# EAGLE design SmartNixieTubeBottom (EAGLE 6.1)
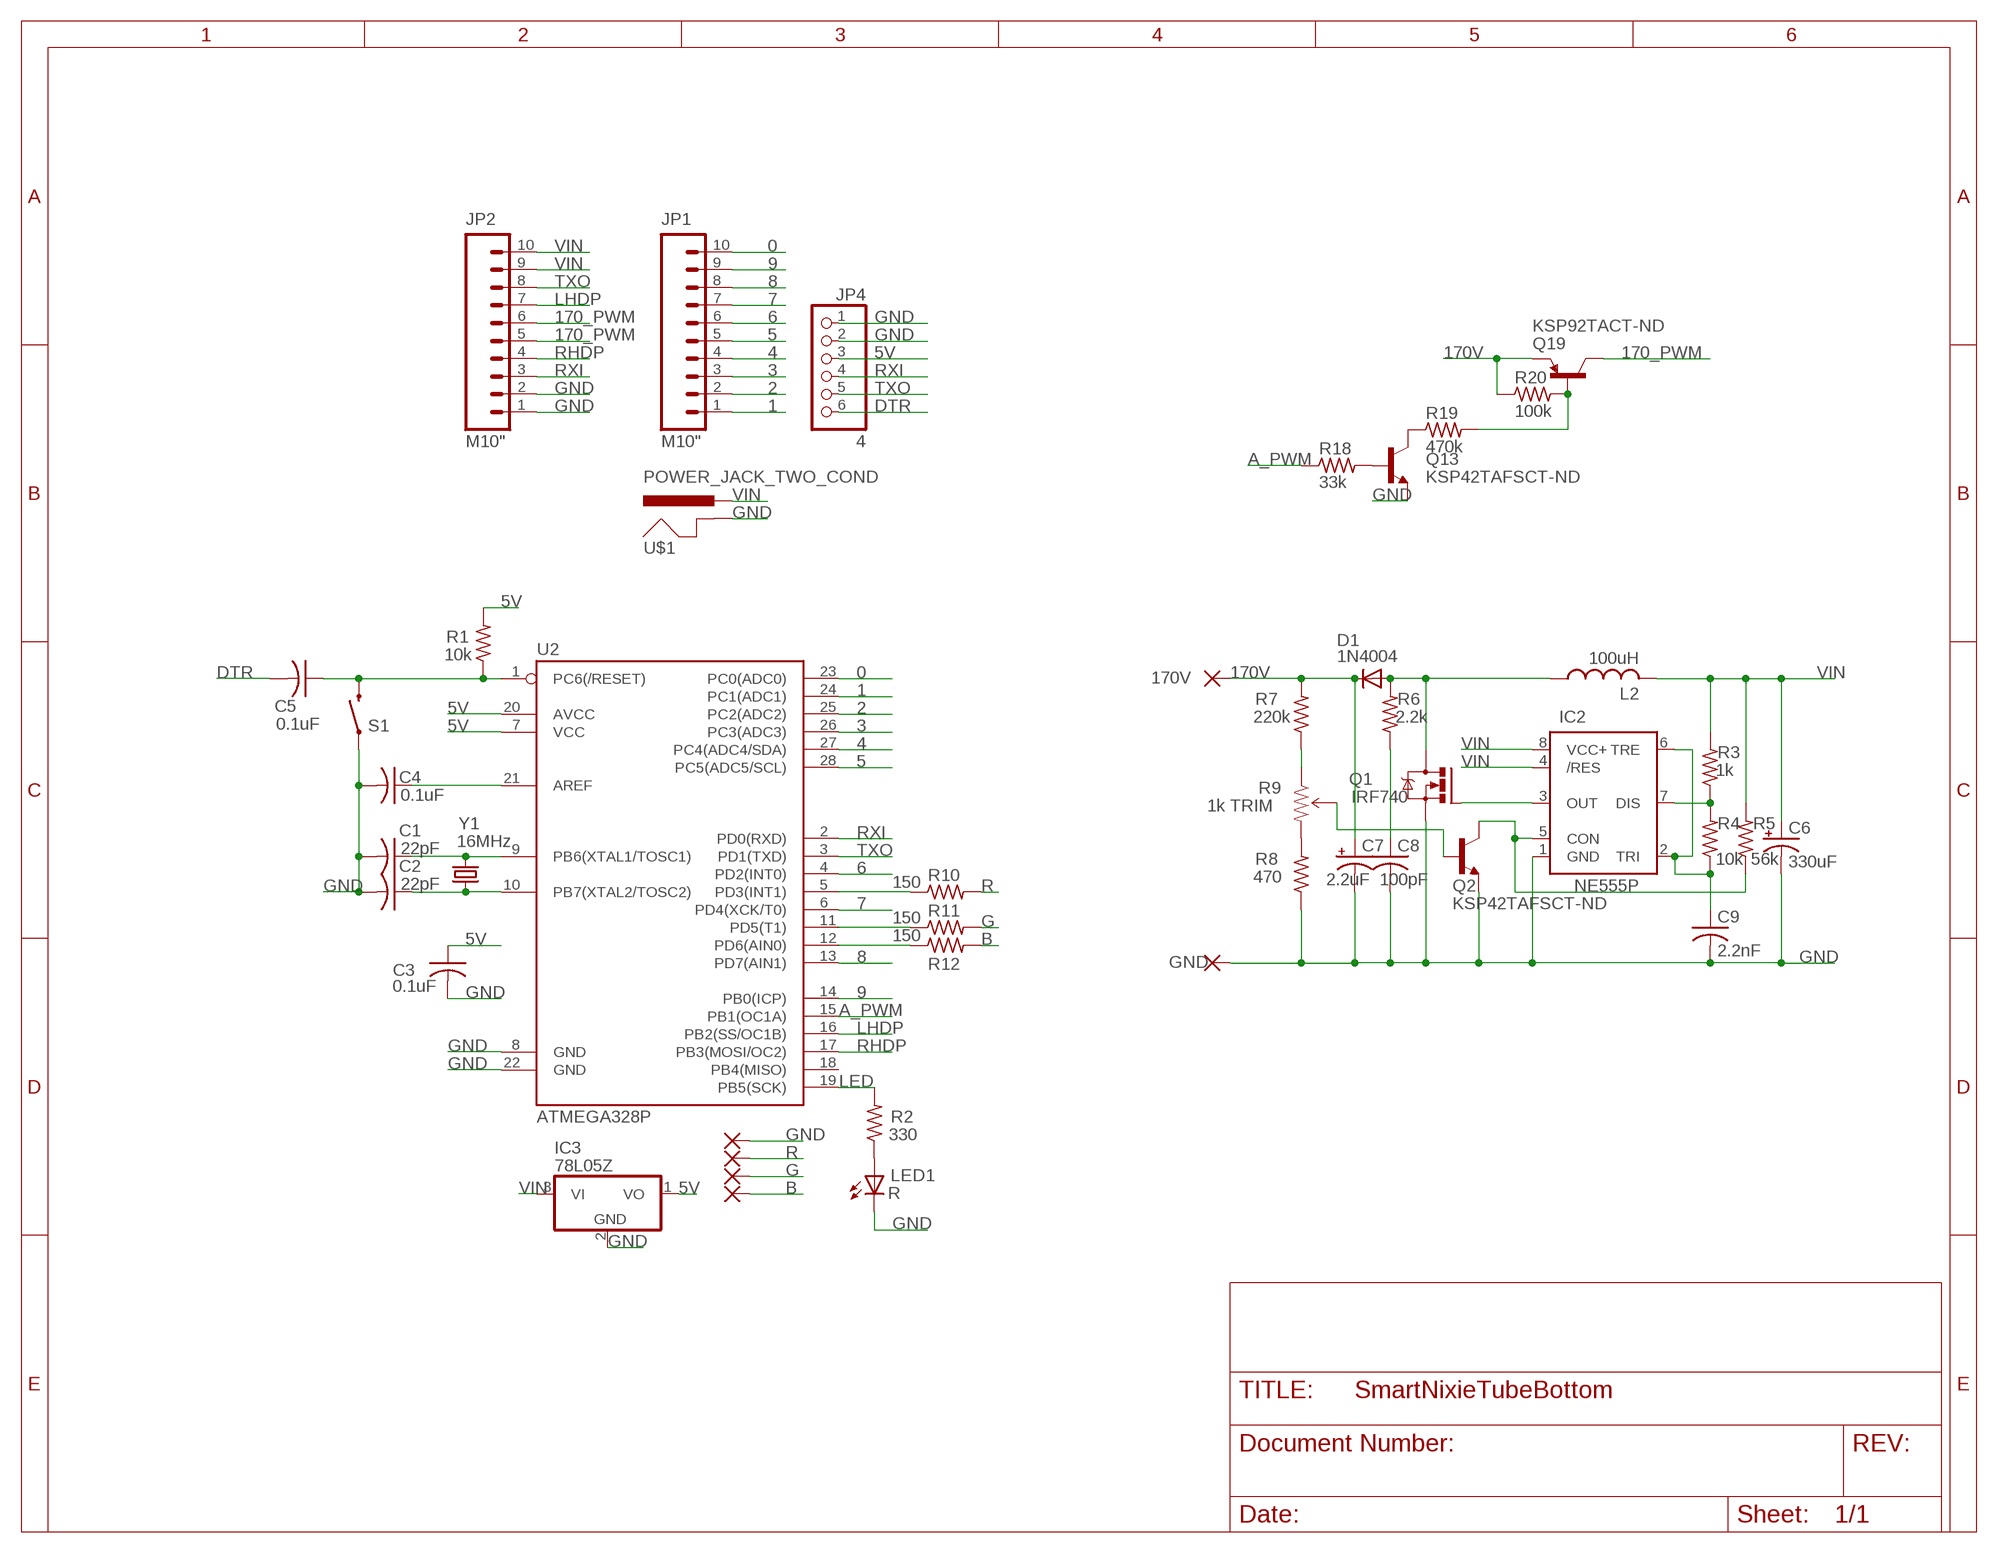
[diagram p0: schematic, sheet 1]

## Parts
C1  22pF  C-US025-024X044  [C025-024X044]
C2  22pF  C-US025-024X044  [C025-024X044]
C3  0.1uF  C-US025-024X044  [C025-024X044]
C4  0.1uF  C-US025-024X044  [C025-024X044]
C5  0.1uF  C-US025-024X044  [C025-024X044]
C6  330uF  CPOL-USE2,5-6E  [E2,5-6E]
C7  2.2uF  CPOL-USE2,5-6E  [E2,5-6E]
C8  100pF  C-US050-025X075  [C050-025X075]
C9  2.2nF  C-US025-025X050  [C025-025X050]
D1  1N4004  [DO41-10]
IC2  NE555P  [DIL-08]
IC3  78L05Z  [TO92]
JP1  M10"  [1X10]
JP2  M10"  [1X10]
JP4  4  PINHD-1X6/90  [1X06/90]
L2  100uH  L-US6000-XXX-RC  [6000-XXXX-RC]
LED1  R  LED5MM  [LED5MM]
PAD1  1  2,15/1,0  [2,15/1,0]
PAD2  2  2,15/1,0  [2,15/1,0]
PAD3  3  2,15/1,0  [2,15/1,0]
PAD4  4  2,15/1,0  [2,15/1,0]
PAD13  GND  1,6/0,8  [1,6/0,8]
PAD14  170V  1,6/0,8  [1,6/0,8]
Q1  IRF740  [TO220BV]
Q2  KSP42TAFSCT-ND  TRANSISTOR_NPNTO-92-AMMO  [TO-92-AMMO]
Q13  KSP42TAFSCT-ND  TRANSISTOR_NPNTO-92-AMMO  [TO-92-AMMO]
Q19  KSP92TACT-ND  TRANSISTOR_PNP  [TO-92-AMMO]
R1  10k  R-US_0204/5  [0204/5]
R2  330  R-US_0204/5  [0204/5]
R3  1k  R-US_0204/5  [0204/5]
R4  10k  R-US_0204/5  [0204/5]
R5  56k  R-US_0204/5  [0204/5]
R6  2.2k  R-US_0204/5  [0204/5]
R7  220k  R-US_0204/5  [0204/5]
R8  470  R-US_0204/5  [0204/5]
R9  1k TRIM  TRIMPOTPTH  [TRIM_POT_PTH]
R10  150  R-US_0204/5  [0204/5]
R11  150  R-US_0204/5  [0204/5]
R12  150  R-US_0204/5  [0204/5]
R18  33k  R-US_0204/5  [0204/5]
R19  470k  R-US_0204/5  [0204/5]
R20  100k  R-US_0204/5  [0204/5]
S1  SWITCH-MOMENTARY-2PTH  [TACTILE-PTH]
U2  ATMEGA328P  ATMEGA328P_PDIP  [DIL28-3]
U$1  POWER_JACK_TWO_COND  [POWER_JACK_TWO_COND]
Y1  16MHz  CRYSTALHC49US  [HC49US]

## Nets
0: JP1.10 U2.23(PC0(ADC0))
1: JP1.1 U2.24(PC1(ADC1))
2: JP1.2 U2.25(PC2(ADC2))
3: JP1.3 U2.26(PC3(ADC3))
4: JP1.4 U2.27(PC4(ADC4/SDA))
5: JP1.5 U2.28(PC5(ADC5/SCL))
5V: C3.1 IC3.1(VO) JP4.3 R1.2 U2.7(VCC) U2.20(AVCC)
6: JP1.6 U2.4(PD2(INT0))
7: JP1.7 U2.6(PD4(XCK/T0))
8: JP1.8 U2.13(PD7(AIN1))
9: JP1.9 U2.14(PB0(ICP))
170_PWM: JP2.5 JP2.6 Q19.3(C)
170V: C7.+ D1.C PAD14.1(P) Q19.1(E) R7.2 R20.1
A_PWM: R18.1 U2.15(PB1(OC1A))
B: PAD4.1(P) R12.2
DTR: C5.2 JP4.6
G: PAD3.1(P) R11.2
GND: C1.2 C2.2 C3.2 C4.2 C6.- C7.- C8.2 C9.2 IC2.1(GND) IC3.2(GND) JP2.1 JP2.2 JP4.1 JP4.2 LED1.K(C) PAD1.1(P) PAD13.1(P) Q1.S Q2.1(E) Q13.1(E) R8.1 S1.1 U2.8(GND) U2.22(GND) U$1.P$1(GNDBREAK)
LED: R2.2 U2.19(PB5(SCK))
LHDP: JP2.7 U2.16(PB2(SS/OC1B))
N$1: C1.1 U2.9(PB6(XTAL1/TOSC1)) Y1.2
N$2: C2.1 U2.10(PB7(XTAL2/TOSC2)) Y1.1
N$3: C4.1 U2.21(AREF)
N$4: LED1.A R2.1
N$5: IC2.3(OUT) Q1.G
N$7: IC2.7(DIS) R3.1 R4.2
N$8: C9.1 IC2.2(TRI) IC2.6(TRE) R4.1
N$9: IC2.5(CON) Q2.3(C) R5.1
N$10: D1.A L2.1 Q1.D R6.2
N$11: C8.1 R6.1
N$12: R8.2 R9.3(CW)
N$13: R7.1 R9.1(CCW)
N$14: Q2.2(B) R9.2(WIPER)
N$15: Q13.2(B) R18.2
N$17: R10.1 U2.5(PD3(INT1))
N$18: R11.1 U2.11(PD5(T1))
N$19: R12.1 U2.12(PD6(AIN0))
N$20: Q13.3(C) R19.1
N$28: Q19.2(B) R19.2 R20.2
R: PAD2.1(P) R10.2
RESET: C5.1 R1.1 S1.3 U2.1(PC6(/RESET))
RHDP: JP2.4 U2.17(PB3(MOSI/OC2))
RXI: JP2.3 JP4.4 U2.2(PD0(RXD))
TXO: JP2.8 JP4.5 U2.3(PD1(TXD))
VIN: C6.+ IC2.4(/RES) IC2.8(VCC+) IC3.3(VI) JP2.9 JP2.10 L2.2 R3.2 R5.2 U$1.P$2(PWR)
Unconnected: U2.18(PB4(MISO))

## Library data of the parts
C1-C5 C8 = rcl:C-US: CAPACITOR, American symbol
C6 C7 = resistor:CPOL-US: POLARIZED CAPACITOR, American symbol
C9 = resistor:C-US: CAPACITOR, American symbol
D1 = diode:1N4004: DIODE
IC2 = SparkFun-AnalogIC:NE555: General purpose bipolar Timer; MF: Arrow Electronics; MPN: NE555N; OC_FARNELL: 1467742; OC_NEWARK: 89K1486
IC3 = linear:78*: Positive VOLTAGE REGULATOR Source: http://cache.national.com/ds/LM/LM78L05.pdf http://www.fairchildsemi.com/ds/LM/LM7805.pdf
JP1 JP2 = SparkFun-Connectors_tyler:M10: Header 10 Standard 10-pin 0.1" header. Use with straight break away headers (SKU : PRT-00116), right angle break away headers (PRT-00553), swiss pins (PRT-00743), machine pins (PRT-00117), and female headers (PRT-00115).
JP4 = pinhead:PINHD-1X6: PIN HEADER
L2 = rcl:L-US: INDUCTOR, American symbol
LED1 = SparkFun-LED:LED: LEDs
PAD1-PAD4 = wirepad:2,15/1,0: THROUGH-HOLE PAD
PAD13 PAD14 = wirepad:1,6/0,8: THROUGH-HOLE PAD
Q1 = transistor-power:IRF740: N-CHANNEL MOS FET
Q2 Q13 = SparkFun-DiscreteSemi:TRANSISTOR_NPN: Generic NPN BJT. MMBT2222 is the common NPN we use. Double check against datasheet- not all devices are the same!
Q19 = SparkFun-DiscreteSemi_tyler:TRANSISTOR_PNP: Generic PNP BJT. Double check pinouts against datasheets- not all devices are the same!
R1-R8 R10-R12 R18-R20 = resistor:R-US_: RESISTOR, American symbol
R9 = SparkFun-Electromechanical:TRIMPOT: Various small potentiometers for "set-and-forget" applications
S1 = SparkFun-Electromechanical:SWITCH-MOMENTARY-2: Various NO switches- pushbuttons, reed, etc
U2 = SparkFun-DigitalIC_tyler:ATMEGA328P_PDIP: uC used in the Arduino 32kb flash, 1k EEPROM, 2k SRAM This is the through-hole version of this chip.
U$1 = SparkFun-Connectors_tyler:POWER_JACK_TWO_COND
Y1 = SparkFun-FreqCtrl:CRYSTAL: Various standard crystals. Proven footprints. Spark Fun Electronics SKU : COM-00534

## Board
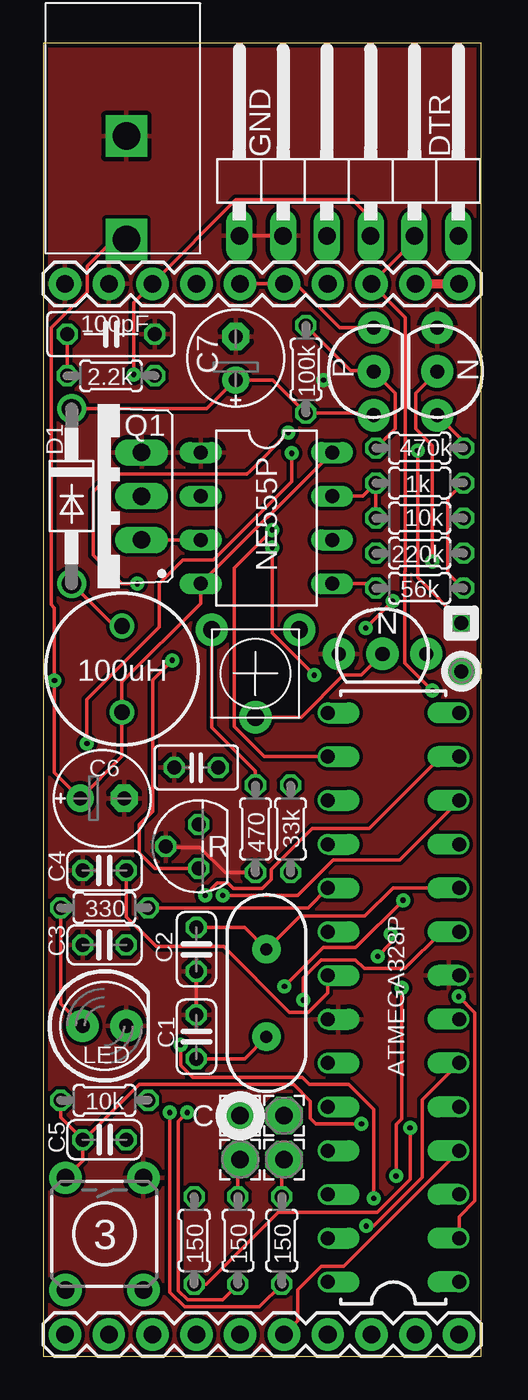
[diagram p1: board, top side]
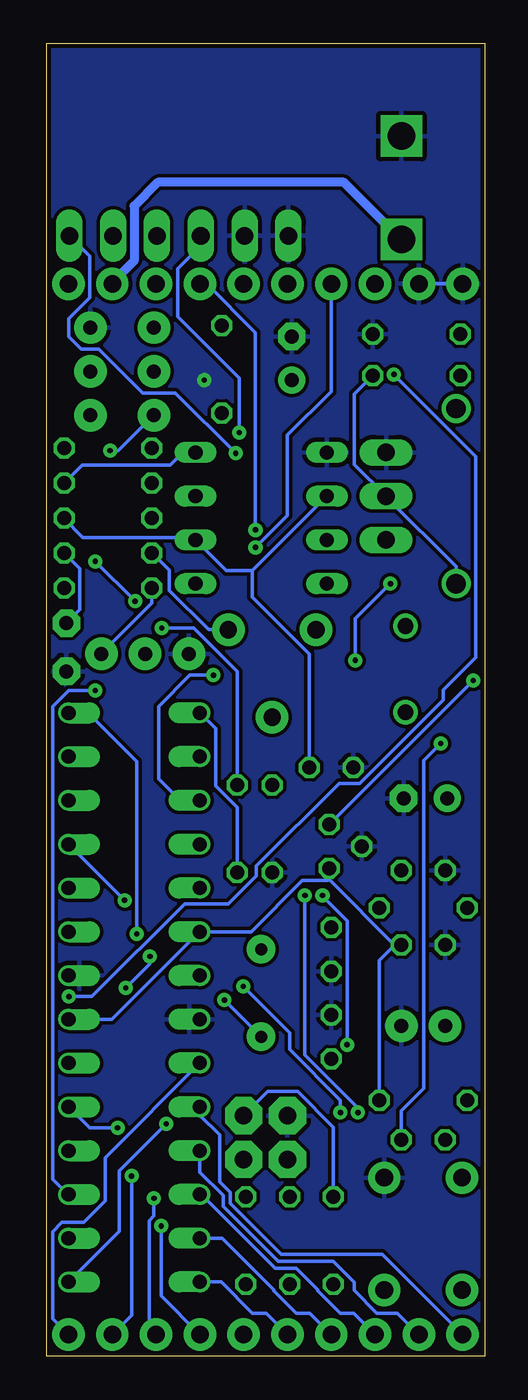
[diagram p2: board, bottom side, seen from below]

Size 25.41 x 76.2 mm. Coordinates in mm from the lower left corner, seen from the top.
Outline: 0,0 25.41,0 25.41,76.2 0,76.2 0,0
Copper layers (1*16): Top 0.035mm / dielectric 1.5mm / Bottom 0.035mm
Design rules: minimum track width 8mil, minimum drill 12mil, track to track 8mil, track to pad 8mil, pad to pad 8mil, via to via 8mil, smd to smd 8mil, copper to edge 10mil, drill to drill 6mil, minimum pad ring 8mil, minimum via ring 10mil, stop-mask expansion 4mil, vias tented up to drill 25mil, thermal gap 10mil

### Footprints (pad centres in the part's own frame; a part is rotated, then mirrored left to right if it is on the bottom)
C025-024X044 = drill 0.813 octagon: 1 -1.27,0; 2 1.27,0
E2,5-6E = drill 0.813 pad 1.575: + -1.27,0 | drill 0.813 pad 1.575 octagon: - 1.27,0
C050-025X075 = drill 0.813 octagon: 1 -2.54,0; 2 2.54,0
C025-025X050 = drill 0.813 octagon: 1 -1.27,0; 2 1.27,0
DO41-10 = drill 1.118: A 5.08,0; C -5.08,0
DIL-08 = drill 0.813 long: 1 -3.81,-3.81; 2 -1.27,-3.81; 3 1.27,-3.81; 4 3.81,-3.81; 5 3.81,3.81; 6 1.27,3.81; 7 -1.27,3.81; 8 -3.81,3.81
TO92 = drill 0.813 octagon: 1 -1.27,0; 2 0,1.905; 3 1.27,0
1X10 = drill 1.016 pad 1.88: 1 0,0; 2 2.54,0; 3 5.08,0; 4 7.62,0; 5 10.16,0; 6 12.7,0; 7 15.24,0; 8 17.78,0; 9 20.32,0; 10 22.86,0
1X06/90 = drill 1.016 long: 1 -6.35,-3.81; 2 -3.81,-3.81; 3 -1.27,-3.81; 4 1.27,-3.81; 5 3.81,-3.81; 6 6.35,-3.81
6000-XXXX-RC = drill 0.9 pad 1.422: 1 -2.5,0; 2 2.5,0
LED5MM = drill 0.813 pad 1.88: A -1.27,0; K 1.27,0
2,15/1,0 = drill 1.016 pad 2.159 octagon: 1 0,0
1,6/0,8 = drill 0.813 pad 1.6 octagon: 1 0,0
TO220BV = drill 1.016 long: D 0,-2.54; G -2.54,-2.54; S 2.54,-2.54
TO-92-AMMO = drill 0.813 pad 1.88: 1 -2.54,0; 2 0,0; 3 2.54,0
0204/5 = drill 0.813 octagon: 1 -2.54,0; 2 2.54,0
TRIM_POT_PTH = drill 1 pad 1.88: 1 -2.54,-2.54; 2 0,2.54; 3 2.54,-2.54
TACTILE-PTH = drill 1.016 pad 1.88: 1 -3.251,2.261; 2 3.251,2.261; 3 -3.251,-2.261; 4 3.251,-2.261
DIL28-3 = drill 0.813 offset: 1 -16.51,-3.81; 2 -13.97,-3.81; 3 -11.43,-3.81; 4 -8.89,-3.81; 5 -6.35,-3.81; 6 -3.81,-3.81; 7 -1.27,-3.81; 8 1.27,-3.81; 9 3.81,-3.81; 10 6.35,-3.81; 11 8.89,-3.81; 12 11.43,-3.81; 13 13.97,-3.81; 14 16.51,-3.81; 15 16.51,3.81; 16 13.97,3.81; 17 11.43,3.81; 18 8.89,3.81; 19 6.35,3.81; 20 3.81,3.81; 21 1.27,3.81; 22 -1.27,3.81; 23 -3.81,3.81; 24 -6.35,3.81; 25 -8.89,3.81; 26 -11.43,3.81; 27 -13.97,3.81; 28 -16.51,3.81
POWER_JACK_TWO_COND = drill 1.6 square: P$1 4.7,6.8; P$2 4.7,0.8
HC49US = drill 0.7 pad 1.651: 1 -2.54,0; 2 2.54,0

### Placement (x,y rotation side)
C1  8.89,18.54 90 top
C2  8.89,23.62 270 top
C3  3.56,23.88 180 top
C4  3.56,28.19 180 top
C5  3.56,12.57 0 top
C6  3.43,32.38 0 top
C7  11.18,57.91 90 top
C8  3.94,59.31 0 top
C9  8.89,34.16 180 top
D1  1.65,49.91 270 top
IC2  12.95,48.64 270 top
IC3  9.02,29.59 90 top
JP1  1.27,1.27 0 top
JP2  1.27,62.23 0 top
JP4  17.73,68.83 0 top
L2  4.57,39.88 270 top
LED1  3.56,19.18 0 top
PAD1  11.43,13.97 0 top
PAD2  13.97,13.97 0 top
PAD3  11.43,11.43 0 top
PAD4  13.97,11.43 0 top
PAD13  24.26,39.75 0 top
PAD14  24.26,42.55 0 top
Q1  3.17,49.91 90 top
Q2  19.68,40.77 0 top
Q13  22.86,57.15 270 top
Q19  19.18,57.15 90 top
R1  3.56,14.86 0 top
R2  3.56,26.04 0 top
R3  21.84,50.67 0 top
R4  21.84,48.64 180 top
R5  21.84,44.58 0 top
R6  3.94,56.9 0 top
R7  21.84,46.61 0 top
R8  12.32,30.61 90 top
R9  12.32,39.62 180 top
R10  8.76,6.73 90 top
R11  11.3,6.73 90 top
R12  13.84,6.73 90 top
R18  14.35,30.61 90 top
R19  21.84,52.7 180 top
R20  15.24,57.28 90 top
S1  3.56,7.11 270 top
U2  20.32,20.83 90 top
U$1  0.13,64.01 0 top
Y1  12.95,21.08 270 top

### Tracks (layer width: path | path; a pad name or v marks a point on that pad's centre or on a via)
0
  Bottom 0.203: U2.23 22,11.53 22,9.02 23.24,7.77 24.51,7.77 25.04,7.24 25.04,2.18 JP1.10
1
  Bottom 0.203: U2.24 16.51,13.99 15.37,12.85 15.37,10.13 14.76,9.53 14.76,8.89 11.79,5.92 5.92,5.92 JP1.1
2
  Bottom 0.203: U2.25 16.51,10.69 15.16,9.35 15.16,8.71 11.96,5.51 8.79,5.51 7.57,4.29 7.57,3.83 6.25,2.52 5.05,2.52 JP1.2
3
  Bottom 0.203: U2.26 16.43,9.4 12.14,5.11 10.92,5.11 9.68,3.86 9.68,3.81 8.38,2.52 7.59,2.52 JP1.3
4
  Bottom 0.203: U2.27 15.21,6.86 12.22,3.86 12.22,3.81 10.92,2.52 10.13,2.52 JP1.4
5
  Bottom 0.203: U2.28 15.27,4.32 13.46,2.52 12.68,2.52 JP1.5
5V  (via drill 0.3)
  Top 0.203: v14.22,53.59 12,51.37 11.81,51.18 3.94,51.18 2.92,50.16 2.92,46.48 4.57,44.83 v5.46,44.83 | IC3.1 6.48,28.32 5.59,29.21 5.59,30.86 6.35,31.62 6.35,39.24 v7.49,40.39
  Bottom 0.203: 9.02,27.66 5.23,23.88 C3.1 5.28,23.8 6.1,22.99 R1.2 | IC3.1 9.02,27.66 | 9.02,27.66 9.09,27.61 10.57,27.61 13.54,24.64 U2.20 16.59,24.59 21.61,19.56 U2.7 | JP4.3 16.46,64.44 17.78,63.12 17.78,60.33 14.22,56.77 v14.22,53.59 | v7.49,40.39 7.49,42.8 v5.46,44.83
6
  Top 0.203: U2.4 17.42,5.23 16.13,5.23 14.76,3.86 14.76,2.06 JP1.6
7  (via drill 0.3)
  Top 0.203: U2.6 22,14.88 22,10.39 19.18,7.57 v18.75,7.57
  Bottom 0.203: v18.75,7.57 18.75,3.5 JP1.7
8  (via drill 0.3)
  Top 0.203: U2.13 23.09,34.8 18.92,30.63 15.62,30.63 13.23,28.25 13.23,27.69 12.7,27.15 11.02,27.15 10.72,27.46 10.11,27.46 v9.4,26.75 | v7.98,18.09 7.98,16.89 8.69,16.18 15.04,16.18 15.44,15.77 17.73,15.77 19.18,14.33 v19.18,9.17
  Bottom 0.203: v9.4,26.75 9.4,26.7 7.98,25.27 v7.98,18.09 | v19.18,9.17 19.18,8.15 19.46,7.87 19.46,1.68 JP1.8
9  (via drill 0.3)
  Top 0.203: v20.17,24.51 20.17,23.98 v19.41,23.22 | v20.8,21.39 20.8,13.79 20.47,13.46 v20.47,10.46
  Bottom 0.203: U2.14 22.99,37.34 20.17,34.52 v20.17,24.51 | v19.41,23.22 19.41,22.78 v20.8,21.39 | v20.47,10.46 20.47,2.39 JP1.9
170_PWM
  Top 0.203: JP2.5 JP2.6 14.05,62.18 14.71,62.18 17.2,59.69 Q19.3
170V  (via drill 0.3)
  Top 0.203: Q19.1 19.05,54.74 R20.1 15.16,54.79 13.31,56.64 C7.+ 11.1,56.59 9.5,54.99 D1.C | PAD14.1 24.26,42.65 21.72,45.19 v21.72,52.55
  Bottom 0.203: R7.2 24.38,46.63 23.47,45.72 23.47,43.33 PAD14.1 | v21.72,52.55 21.23,52.55 Q19.1
A_PWM
  Bottom 0.203: R18.1 14.35,31.85 15.6,33.1 15.6,36.42 U2.15
B
  Top 0.203: R12.2 13.84,11.3 PAD4.1
DTR  (via drill 0.3)
  Top 0.203: v2.54,35.56 2.54,38.12 6.73,42.32 6.73,44.83 8.1,46.2 9.88,46.2 14.43,50.75 v14.43,52.4
  Bottom 0.203: C5.2 4.83,14.25 3.53,15.54 3.53,34.57 v2.54,35.56 | v14.43,52.4 17.93,55.91 19.84,55.91 22.38,58.45 23.39,58.45 24.11,59.16 24.11,60.22 22.89,61.44 22.89,63.83 JP4.6
G
  Top 0.203: R11.2 11.3,11.3 PAD3.1
GND  (via drill 0.3)
  Top 0.203: JP4.2 JP4.1 | R8.1 10.57,28.07 9.09,29.54 7.19,29.54 IC3.2 | C2.2 C1.2
  Bottom 0.203: JP2.2 JP2.1
  other vias: 16.26,56.64
  pour Bottom (isolate 0.203): 0,0 25.4,0 25.4,76.2 0,76.2
  pour Top (isolate 0.203): 0,0 25.4,0 25.4,76.2 0,76.2
LED
  Top 0.203: R2.2 15.37,26.04 U2.19
LHDP  (via drill 0.3)
  Top 0.203: U2.16 12.83,34.8 11.07,36.55 11.07,45.74 v13.28,47.95
  Bottom 0.203: v13.28,47.95 13.28,59.41 16.1,62.23 JP2.7
N$1  (via drill 0.3)
  Top 0.203: C1.1 11.68,17.27 Y1.2 | U2.9 23.11,24.64 20.98,22.5 18.62,22.5 18.11,23.01 16.13,23.01 15.09,21.97 v15.09,20.68
  Bottom 0.203: Y1.2 v15.09,20.68
N$2
  Top 0.203: C2.1 11.68,24.89 Y1.1 13.03,23.67 14.91,25.55 18.67,25.55 20.3,27.18 U2.10
N$3
  Top 0.203: C4.1 4.83,25.5 6.55,23.77 10.46,23.77 14.28,19.96 15.39,19.96 16.51,21.08 U2.21
N$4
  Top 0.203: R2.1 1.02,20.45 LED1.A
N$5
  Top 0.203: Q1.G IC2.3
N$7
  Top 0.203: IC2.7 18.54,49.91 R3.1 R4.2
N$8
  Bottom 0.203: C9.1 10.16,40.77 13.46,44.07 13.46,45.59 | 13.46,45.59 IC2.2 | R4.1 24.41,48.64 23.29,47.52 16.94,47.52 16.84,47.42 IC2.6 14.99,45.59 13.46,45.59
N$9
  Top 0.203: IC2.5 19.05,44.83 R5.1
  Bottom 0.203: R5.1 19.3,43.71 22.23,40.79 Q2.3
N$10
  Top 0.203: D1.A 4.09,42.39 4.57,42.39 L2.1
  Bottom 0.203: R6.2 7.54,55.83 7.54,51.74 Q1.D 5.66,49.84 1.65,45.82 D1.A
N$11
  Top 0.203: C8.1 R6.1
N$12
  Top 0.203: R8.2 12.32,33.96 9.78,36.5 R9.3
N$13
  Bottom 0.203: R7.1 19.3,46.63 18.29,45.62 18.29,44.45 16,42.16 R9.1
N$14
  Top 0.203: R9.2 14.96,37.08 17.4,39.52 18.44,39.52 Q2.2
N$15  (via drill 0.3)
  Top 0.203: v20.27,43.81 v18.72,42.27 | v22.58,46.13 22.58,52.86 21.61,53.82 21.61,55.91 Q13.2
  Bottom 0.203: R18.2 14.35,39.75 16.87,42.27 v18.72,42.27 | v22.58,46.13 v20.27,43.81
N$17  (via drill 0.3)
  Top 0.203: R10.1 9.47,4.19 13.64,8.36 19.38,8.36 21.29,10.26 v21.29,13.26
  Bottom 0.203: v21.29,13.26 22.91,13.26 U2.5
N$18  (via drill 0.3)
  Top 0.203: R11.1 11.33,4.19 10.41,3.28 8.38,3.28 7.85,3.81 7.85,13.64 v8.36,14.15 | v13.99,21.46 16.26,23.72 18.14,23.72 v20.88,26.47
  Bottom 0.203: v8.36,14.15 8.36,14.86 11.3,17.8 11.3,18.77 v13.99,21.46 | U2.11 v20.88,26.47
N$19  (via drill 0.3)
  Top 0.203: R12.1 13.87,4.19 12.55,2.87 8.2,2.87 7.34,3.73 v7.34,14.15 | v10.41,26.75 14.78,26.75 16.84,28.8 20.68,28.8 U2.12
  Bottom 0.203: v7.34,14.15 7.34,14.43 10.41,17.5 v10.41,26.75
N$20
  Top 0.203: R19.1 24.38,53.09 Q13.3
N$28
  Top 0.203: R19.2 20.42,53.82 20.42,55.91 Q19.2 19.1,57.2 17.86,57.2 R20.2
R
  Bottom 0.203: R10.2 8.76,13.28 10.85,15.37 12.57,15.37 PAD2.1
RESET  (via drill 0.3)
  Top 0.203: C5.1 2.29,11.35 S1.3 | R1.1 1.02,13.87 2.23,12.65 C5.1 | v18.47,13.49 15.82,13.49 15.49,13.82 15.49,14.81 14.53,15.77 5.56,15.77 2.39,12.6 C5.1
  Bottom 0.203: U2.1 21.18,7.26 21.18,10.77 v18.47,13.49
RHDP  (via drill 0.3)
  Top 0.203: v15.72,39.52 13.28,41.96 v13.28,46.94
  Bottom 0.203: U2.17 17.65,32.26 18.9,33.5 18.9,37.72 17.09,39.52 v15.72,39.52 | v13.28,46.94 11.43,48.79 11.43,53.44 8.89,55.98 JP2.4 8.89,62.28
RXI  (via drill 0.3)
  Top 0.203: U2.2 24.13,8.1 25.04,9.02 25.04,19.94 v24.11,20.88 | v5.26,56.97 5.26,61.14 JP2.3 6.38,62.31 11.18,67.11 17.93,67.11 19,66.04 JP4.4
  Bottom 0.203: v24.11,20.88 22.78,20.88 17.4,26.26 14.86,26.26 13.23,27.89 13.23,28.45 8.43,33.25 7.24,33.25 2.39,38.1 2.39,38.66 0.51,40.54 0.51,52.22 v5.26,56.97
TXO  (via drill 0.3)
  Top 0.203: v22.58,38.63 20.98,40.23 20.98,45.54 21.01,45.57 21.01,60.27 JP2.8 19.1,62.31 21.54,64.75 JP4.5
  Bottom 0.203: U2.3 24.13,9.37 25.04,10.29 25.04,37.72 24.13,38.63 v22.58,38.63
VIN  (via drill 0.3)
  Top 0.203: R5.2 24.38,44.55 23.47,45.47 23.47,49.76 R3.2 | IC2.8 IC2.4 9.14,43.69 4.57,39.12 L2.2 4.57,34.8 C6.+ 0.66,33.88 v0.66,39.22 0.66,43.43 0.48,43.61 0.48,59.69 1.78,60.98 1.8,60.98 2.56,61.75 2.56,63.27 4.09,64.8 4.83,64.8
  Top 0.508: 4.83,64.8 U$1.P$2 | JP2.9 JP2.10
  Bottom 0.203: IC2.8 17.5,52.45 18.24,51.71 23.34,51.71 R3.2 | 21.59,62.31 JP2.9 | v0.66,39.22 IC3.3
  Bottom 0.508: 21.59,62.31 20.32,63.58 20.32,66.75 18.95,68.12 8.15,68.12 4.85,64.82 U$1.P$2

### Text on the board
tPlace: GND | DTR | 100pF | N | P | N | R | LED | C | 3

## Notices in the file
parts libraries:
SparkFun-DigitalIC_tyler: Licensing: CC v3.0 Share-Alike You are welcome to use this library for commercial purposes.
